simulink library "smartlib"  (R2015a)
settings: Solver=ode45  StartTime=0.0  StopTime=10.0  RelTol=1e-3
undefined symbols (not defined in the file or in its folder): annualChangeOfCostPerKwhFromUtility, batteryCostPerKwh, batterySize, compensationPerKwhSoldToBattery, costPerKwhBoughtFromBattery, costPerKwhFromUtility, csvread, numberOfHouses, oneTimeCost, randi, solarPanelEfficiency
libraries: simulink x7

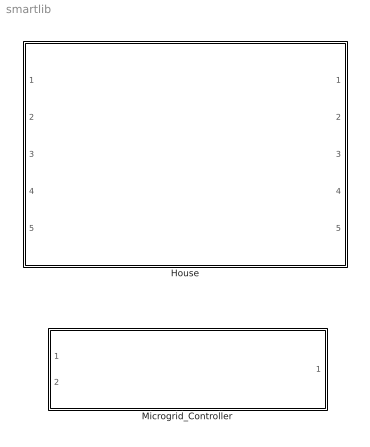
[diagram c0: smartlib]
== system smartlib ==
  House : Subsystem
  Microgrid_Controller : Subsystem

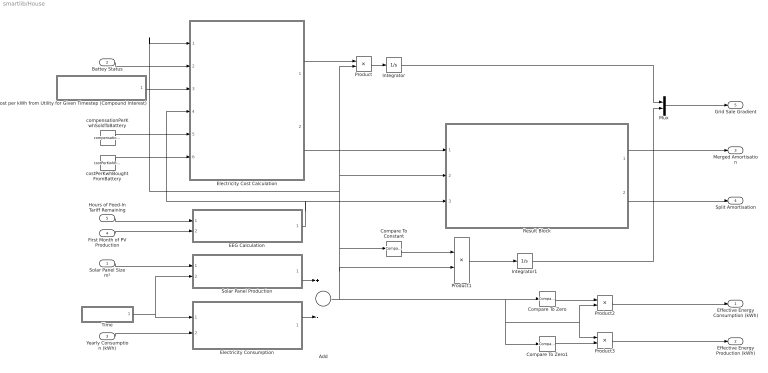
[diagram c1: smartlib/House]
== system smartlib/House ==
  Solar Panel Size m² : Inport
  Battey Status : Inport  Port=2
  Yearly Consumption (kWh) : Inport  Port=3
  First Month of PV Production : Inport  Port=4
  Hours of Feed-In Tariff Remaining : Inport  Port=5
  Add : Sum  Inputs=+-
  Compare To Constant : simulink/Logic and Bit Operations/Compare To Constant  relop=>=  const=0  OutDataTypeStr=boolean
  Compare To Zero : simulink/Logic and Bit Operations/Compare To Zero  relop=<  OutDataTypeStr=boolean
  Compare To Zero1 : simulink/Logic and Bit Operations/Compare To Zero  relop=>=  OutDataTypeStr=boolean
  Cost per kWh from Utility for Given Timestep (Compound Interest) : Subsystem
  EEG Calculation : Subsystem
  Electricity Consumption : Subsystem
  Electricity Cost Calculation : MATLAB Function  TreatAsAtomicUnit=on
  Integrator : Integrator
  Integrator1 : Integrator
  Mux : Mux  Inputs=2
  Product{,1..3} (4 alike) : Product
  Result Block : Subsystem
  Solar Panel Production : Subsystem
  Time : Subsystem
  compensationPerKwhSoldToBattery : Constant  Value=compensationPerKwhSoldToBattery
  costPerKwhBoughtFromBattery : Constant  Value=costPerKwhBoughtFromBattery
  Effective Energy Consumption (kWh) : Outport
  Effective Energy Production (kWh) : Outport  Port=2
  Merged Amortisation : Outport  Port=3
  Split Amortisation : Outport  Port=4
  Grid Sale Gradient : Outport  Port=5
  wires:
  Time/1(Time in Hours % 8760) -> Solar Panel Production/2(Hour of Year), Electricity Consumption/1(Hour of Year)
  Solar Panel Size m²/1 -> Solar Panel Production/1(Solar Panel Size (m²))
  Yearly Consumption (kWh)/1 -> Electricity Consumption/2(Yearly Consumption (kWh))
  Product/1 -> Integrator/1
  Compare To Constant/1 -> Product1/1
  Product1/1 -> Integrator1/1
  Product2/1 -> Effective Energy Consumption (kWh)/1
  Product3/1 -> Effective Energy Production (kWh)/1
  Compare To Zero1/1 -> Product3/2
  Compare To Zero/1 -> Product2/1
  Battey Status/1 -> Electricity Cost Calculation/2(batteryStatus)
  costPerKwhBoughtFromBattery/1 -> Electricity Cost Calculation/6(internalBuyPrice)
  Cost per kWh from Utility for Given Timestep (Compound Interest)/1(Cost for kWh from Utility at Timestep) -> Electricity Cost Calculation/3(buyPrice)
  Electricity Cost Calculation/1(gridsaleAmount) -> Product/1
  Electricity Consumption/1(Consumtion kWh) -> Add/2
  Solar Panel Production/1(Solar Panel Production (kWh)) -> Add/1
  Add/1 -> Compare To Zero1/1, Product3/1, Product2/2, Compare To Zero/1, Product/2, Result Block/2(Effective Consumption / Production (kWh)), Electricity Cost Calculation/1(kWh), Compare To Constant/1, Product1/2
  EEG Calculation/1(Applcable Feed-In Tariff) -> Electricity Cost Calculation/4(sellPrice), Result Block/3(Applicable Feed-In Tariff (EUR))
  Result Block/1(House Result Merged) -> Merged Amortisation/1
  Result Block/2(House Result Split) -> Split Amortisation/1
  Integrator/1 -> Mux/1
  Integrator1/1 -> Mux/2
  Mux/1 -> Grid Sale Gradient/1
  Electricity Cost Calculation/2(cost) -> Result Block/1(Effective Cost of Electricity for Timestep (EUR))
  Hours of Feed-In Tariff Remaining/1 -> EEG Calculation/1(Hours of Feed-In Tariff Remaining)
  First Month of PV Production/1 -> EEG Calculation/2(First Month of PV Production)
  compensationPerKwhSoldToBattery/1 -> Electricity Cost Calculation/5(internalSellPrice)

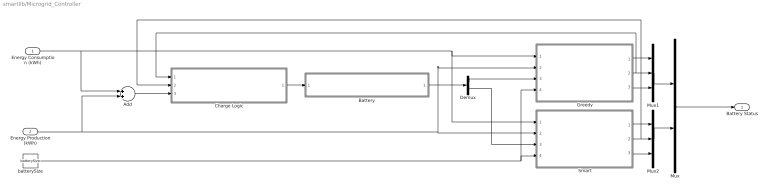
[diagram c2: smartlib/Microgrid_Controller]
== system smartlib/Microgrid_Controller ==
  Energy Consumption (kWh) : Inport
  Energy Production (kWh) : Inport  Port=2
  Add : Sum
  Battery : Subsystem
  Charge Logic : Subsystem
  Demux : Demux  Outputs=2
  Greedy : MATLAB Function  TreatAsAtomicUnit=on
  Mux : Mux  Inputs=2
  Mux1 : Mux  Inputs=3
  Mux2 : Mux  Inputs=3
  Smart : MATLAB Function  TreatAsAtomicUnit=on
  batterySize : Constant  Value=batterySize
  Battery Status : Outport
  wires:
  Charge Logic/1(Charge (kw/h)) -> Battery/1(Charge Amount (kWh))
  Mux/1 -> Battery Status/1
  batterySize/1 -> Smart/4(batterySize), Greedy/4(batterySize)
  Add/1 -> Charge Logic/3(Net Energy Amount (kWh))
  Demux/2 -> Smart/3(currentBatteryCharge)
  Demux/1 -> Greedy/3(currentBatteryCharge)
  Energy Consumption (kWh)/1 -> Greedy/1(Consumption), Smart/1(Consumption), Add/1
  Energy Production (kWh)/1 -> Smart/2(Production), Greedy/2(Production), Add/2
  Greedy/2(p2) -> Mux1/2, Charge Logic/1(Internal Trade Percentage - Greedy)
  Greedy/3(p3) -> Mux1/3
  Greedy/1(p1) -> Mux1/1
  Mux1/1 -> Mux/1
  Smart/1(p1) -> Mux2/1
  Smart/2(p2) -> Charge Logic/2(Internal Trade Percentage - Smart), Mux2/2
  Smart/3(p3) -> Mux2/3
  Mux2/1 -> Mux/2
  Battery/1(Current Battery Charge (kWh)) -> Demux/1

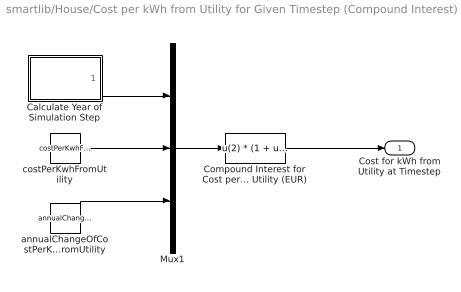
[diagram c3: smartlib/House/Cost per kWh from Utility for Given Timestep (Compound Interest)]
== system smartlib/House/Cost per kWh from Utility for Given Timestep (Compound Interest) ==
  Calculate Year of Simulation Step : Subsystem
  Compound Interest for Cost per kWh from Utility (EUR) : Fcn  Expr=u(2) * (1 + u(3) / 100) ^ u(1)
  Mux1 : Mux  Inputs=3
  annualChangeOfCostPerKwhFromUtility : Constant  Value=annualChangeOfCostPerKwhFromUtility
  costPerKwhFromUtility : Constant  Value=costPerKwhFromUtility
  Cost for kWh from Utility at Timestep : Outport
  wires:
  Mux1/1 -> Compound Interest for Cost per kWh from Utility (EUR)/1
  annualChangeOfCostPerKwhFromUtility/1 -> Mux1/3
  Calculate Year of Simulation Step/1(Out1) -> Mux1/1
  Compound Interest for Cost per kWh from Utility (EUR)/1 -> Cost for kWh from Utility at Timestep/1
  costPerKwhFromUtility/1 -> Mux1/2

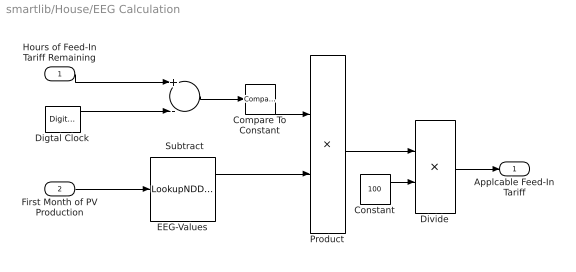
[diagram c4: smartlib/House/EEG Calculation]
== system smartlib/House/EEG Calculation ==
  Hours of Feed-In Tariff Remaining : Inport
  First Month of PV Production : Inport  Port=2
  Compare To Constant : simulink/Logic and Bit Operations/Compare To Constant  relop=>=  const=0  OutDataTypeStr=boolean
  Constant : Constant  Value=100
  Digtal Clock : DigitalClock
  Divide : Product  Inputs=*/
  EEG-Values : LookupNDDirect  NumberOfTableDimensions=1  Table=csvread('raw_data/feed-in_tariff_data.csv');  DiagnosticForOutOfRangeInput=Error
  Product : Product
  Subtract : Sum  Inputs=+-
  Applcable Feed-In Tariff : Outport
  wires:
  First Month of PV Production/1 -> EEG-Values/1
  Hours of Feed-In Tariff Remaining/1 -> Subtract/1
  Digtal Clock/1 -> Subtract/2
  Subtract/1 -> Compare To Constant/1
  Compare To Constant/1 -> Product/1
  EEG-Values/1 -> Product/2
  Divide/1 -> Applcable Feed-In Tariff/1
  Product/1 -> Divide/1
  Constant/1 -> Divide/2

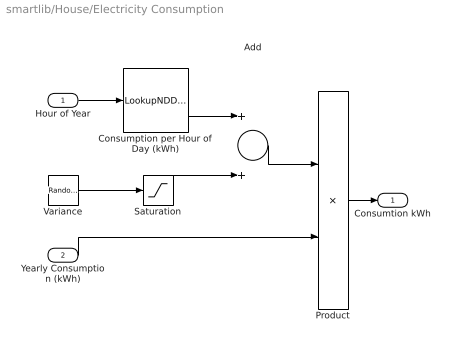
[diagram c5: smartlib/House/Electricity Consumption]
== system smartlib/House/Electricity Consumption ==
  Hour of Year : Inport
  Yearly Consumption (kWh) : Inport  Port=2
  Add : Sum
  Consumption per Hour of Day (kWh) : LookupNDDirect  NumberOfTableDimensions=1  Table=csvread('raw_data/netherlands_consumption_e1a.csv');  DiagnosticForOutOfRangeInput=Error
  Product : Product
  Saturation : Saturate  UpperLimit=5*10e-5  LowerLimit=-5*10e-5
  Variance : RandomNumber  Variance=0.00000000013014  Seed=randi(66666);  SampleTime=1
  Consumtion kWh : Outport
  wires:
  Add/1 -> Product/1
  Consumption per Hour of Day (kWh)/1 -> Add/1
  Hour of Year/1 -> Consumption per Hour of Day (kWh)/1
  Yearly Consumption (kWh)/1 -> Product/2
  Product/1 -> Consumtion kWh/1
  Variance/1 -> Saturation/1
  Saturation/1 -> Add/2

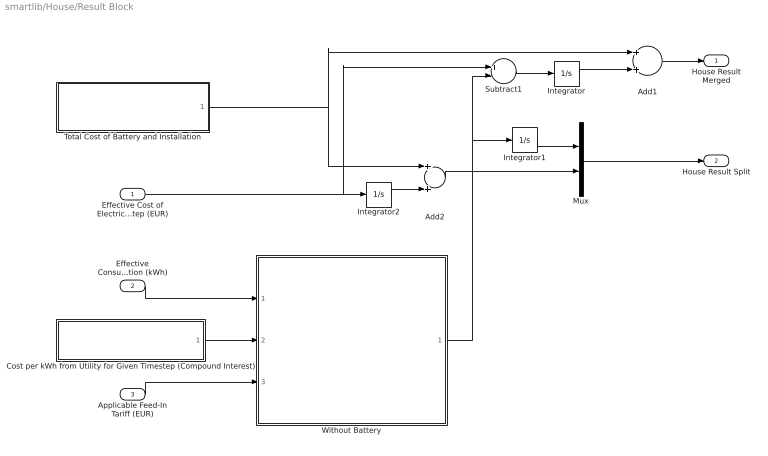
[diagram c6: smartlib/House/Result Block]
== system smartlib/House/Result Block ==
  Effective Cost of Electricity for Timestep (EUR) : Inport
  Effective Consumption / Production (kWh) : Inport  Port=2
  Applicable Feed-In Tariff (EUR) : Inport  Port=3
  Add1 : Sum
  Add2 : Sum
  Cost per kWh from Utility for Given Timestep (Compound Interest) : Subsystem
  Integrator : Integrator
  Integrator1 : Integrator
  Integrator2 : Integrator
  Mux : Mux  Inputs=2
  Subtract1 : Sum  Inputs=+-
  Total Cost of Battery and Installation : Subsystem
  Without Battery : Subsystem
  House Result Merged : Outport
  House Result Split : Outport  Port=2
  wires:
  Applicable Feed-In Tariff (EUR)/1 -> Without Battery/3(Sell Price to Utility (EUR))
  Subtract1/1 -> Integrator/1
  Effective Cost of Electricity for Timestep (EUR)/1 -> Subtract1/1, Integrator2/1
  Add1/1 -> House Result Merged/1
  Effective Consumption / Production (kWh)/1 -> Without Battery/1(Effective Consumption / Production (kWh))
  Integrator/1 -> Add1/2
  Mux/1 -> House Result Split/1
  Integrator1/1 -> Mux/1
  Integrator2/1 -> Add2/2
  Add2/1 -> Mux/2
  Total Cost of Battery and Installation/1(Total Cost of Battery and Installation) -> Add1/1, Add2/1
  Cost per kWh from Utility for Given Timestep (Compound Interest)/1(Cost per kWh from Utility at Timestep) -> Without Battery/2(Cost per kWh from Utility (EUR))
  Without Battery/1(Result EUR) -> Integrator1/1, Subtract1/2

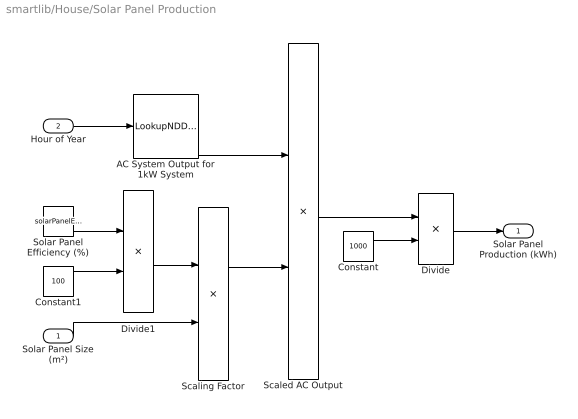
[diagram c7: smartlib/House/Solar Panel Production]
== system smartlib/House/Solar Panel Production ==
  Solar Panel Size (m²) : Inport
  Hour of Year : Inport  Port=2
  AC System Output for 1kW System : LookupNDDirect  NumberOfTableDimensions=1  Table=csvread('raw_data/pvwatts_data_1kwp.csv');  DiagnosticForOutOfRangeInput=Error
  Constant : Constant  Value=1000
  Constant1 : Constant  Value=100
  Divide : Product  Inputs=*/
  Divide1 : Product  Inputs=*/
  Scaled AC Output : Product
  Scaling Factor : Product
  Solar Panel Efficiency (%) : Constant  Value=solarPanelEfficiency
  Solar Panel Production (kWh) : Outport
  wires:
  Solar Panel Efficiency (%)/1 -> Divide1/1
  Scaling Factor/1 -> Scaled AC Output/2
  AC System Output for 1kW System/1 -> Scaled AC Output/1
  Solar Panel Size (m²)/1 -> Scaling Factor/2
  Hour of Year/1 -> AC System Output for 1kW System/1
  Scaled AC Output/1 -> Divide/1
  Constant/1 -> Divide/2
  Divide/1 -> Solar Panel Production (kWh)/1
  Constant1/1 -> Divide1/2
  Divide1/1 -> Scaling Factor/1

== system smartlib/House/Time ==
  Digtal Clock : DigitalClock
  Hours in a Year : Constant  Value=8760
  Modulo : Math  Operator=mod
  Time in Hours % 8760 : Outport
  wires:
  Digtal Clock/1 -> Modulo/1
  Hours in a Year/1 -> Modulo/2
  Modulo/1 -> Time in Hours % 8760/1

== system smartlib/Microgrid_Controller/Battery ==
  Charge Amount (kWh) : Inport
  Battery : Integrator
  To Workspace : ToWorkspace  VariableName=neighbourhood_battery_charge_over_time  SaveFormat=Timeseries  SampleTime=-1
  Current Battery Charge (kWh) : Outport
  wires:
  Battery/1 -> Current Battery Charge (kWh)/1, To Workspace/1
  Charge Amount (kWh)/1 -> Battery/1

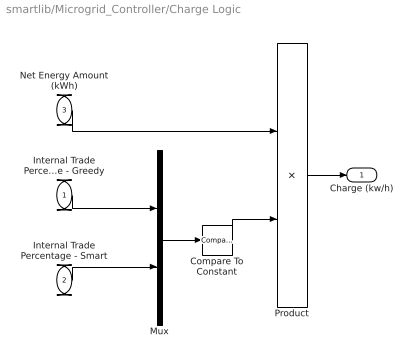
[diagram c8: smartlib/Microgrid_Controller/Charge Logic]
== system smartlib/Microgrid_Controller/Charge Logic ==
  Internal Trade Percentage - Greedy : Inport
  Internal Trade Percentage - Smart : Inport  Port=2
  Net Energy Amount (kWh) : Inport  Port=3
  Compare To Constant : simulink/Logic and Bit Operations/Compare To Constant  relop===  const=1  OutDataTypeStr=boolean
  Mux : Mux  Inputs=2
  Product : Product
  Charge (kw/h) : Outport
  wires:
  Net Energy Amount (kWh)/1 -> Product/1
  Product/1 -> Charge (kw/h)/1
  Internal Trade Percentage - Greedy/1 -> Mux/1
  Mux/1 -> Compare To Constant/1
  Internal Trade Percentage - Smart/1 -> Mux/2
  Compare To Constant/1 -> Product/2

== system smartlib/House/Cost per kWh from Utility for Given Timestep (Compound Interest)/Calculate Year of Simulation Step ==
  Digital Clock : DigitalClock
  Fcn : Fcn  Expr=floor(u/8760)
  Out1 : Outport
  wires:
  Fcn/1 -> Out1/1
  Digital Clock/1 -> Fcn/1

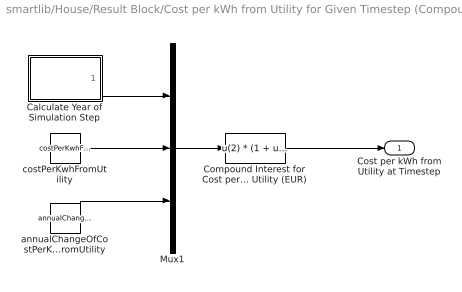
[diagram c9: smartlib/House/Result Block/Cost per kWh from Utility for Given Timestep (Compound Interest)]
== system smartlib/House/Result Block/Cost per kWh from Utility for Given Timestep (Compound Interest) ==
  Calculate Year of Simulation Step : Subsystem
  Compound Interest for Cost per kWh from Utility (EUR) : Fcn  Expr=u(2) * (1 + u(3) / 100) ^ u(1)
  Mux1 : Mux  Inputs=3
  annualChangeOfCostPerKwhFromUtility : Constant  Value=annualChangeOfCostPerKwhFromUtility
  costPerKwhFromUtility : Constant  Value=costPerKwhFromUtility
  Cost per kWh from Utility at Timestep : Outport
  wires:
  Mux1/1 -> Compound Interest for Cost per kWh from Utility (EUR)/1
  annualChangeOfCostPerKwhFromUtility/1 -> Mux1/3
  Calculate Year of Simulation Step/1(Out1) -> Mux1/1
  Compound Interest for Cost per kWh from Utility (EUR)/1 -> Cost per kWh from Utility at Timestep/1
  costPerKwhFromUtility/1 -> Mux1/2

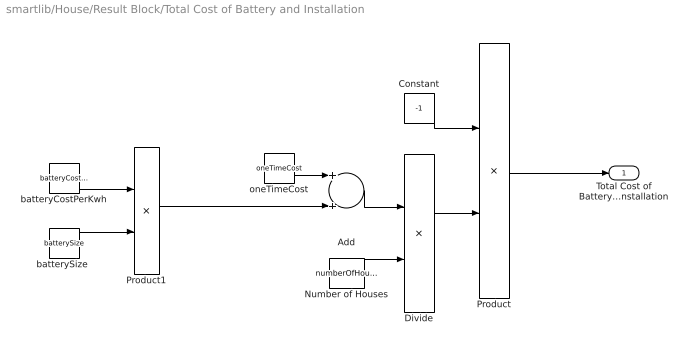
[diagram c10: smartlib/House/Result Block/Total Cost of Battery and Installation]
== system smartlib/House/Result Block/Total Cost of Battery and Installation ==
  Add : Sum
  Constant : Constant  Value=-1
  Divide : Product  Inputs=*/
  Number of Houses : Constant  Value=numberOfHouses
  Product : Product
  Product1 : Product
  batteryCostPerKwh : Constant  Value=batteryCostPerKwh
  "batterySize " : Constant  Value=batterySize
  oneTimeCost : Constant  Value=oneTimeCost
  Total Cost of Battery and Installation : Outport
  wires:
  Constant/1 -> Product/1
  oneTimeCost/1 -> Add/1
  Number of Houses/1 -> Divide/2
  Add/1 -> Divide/1
  Divide/1 -> Product/2
  "batterySize "/1 -> Product1/2
  Product/1 -> Total Cost of Battery and Installation/1
  batteryCostPerKwh/1 -> Product1/1
  Product1/1 -> Add/2

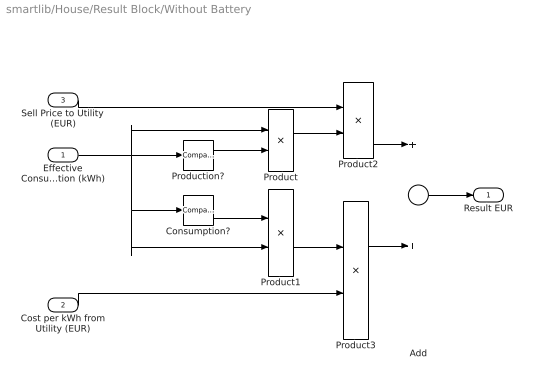
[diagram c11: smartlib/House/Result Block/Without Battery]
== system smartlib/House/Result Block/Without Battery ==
  Effective Consumption / Production (kWh) : Inport
  Cost per kWh from Utility (EUR) : Inport  Port=2
  Sell Price to Utility (EUR) : Inport  Port=3
  Add : Sum
  Consumption? : simulink/Logic and Bit Operations/Compare To Zero  relop=<  OutDataTypeStr=boolean
  Product{,1..3} (4 alike) : Product
  Production? : simulink/Logic and Bit Operations/Compare To Zero  relop=>=  OutDataTypeStr=boolean
  Result EUR : Outport
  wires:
  Effective Consumption / Production (kWh)/1 -> Product/1, Product1/2, Consumption?/1, Production?/1
  Consumption?/1 -> Product1/1
  Production?/1 -> Product/2
  Product/1 -> Product2/2
  Sell Price to Utility (EUR)/1 -> Product2/1
  Product1/1 -> Product3/1
  Cost per kWh from Utility (EUR)/1 -> Product3/2
  Product3/1 -> Add/2
  Product2/1 -> Add/1
  Add/1 -> Result EUR/1

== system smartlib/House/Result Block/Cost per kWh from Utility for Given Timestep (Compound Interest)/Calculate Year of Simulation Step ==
  Digital Clock : DigitalClock
  Fcn : Fcn  Expr=floor(u/8760)
  Out1 : Outport
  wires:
  Fcn/1 -> Out1/1
  Digital Clock/1 -> Fcn/1

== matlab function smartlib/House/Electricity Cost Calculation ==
function [gridsaleAmount, cost]  = costCalculation(kWh, batteryStatus, buyPrice, sellPrice, internalSellPrice, internalBuyPrice)


cost = zeros(numel(batteryStatus)/3 , 1);
gridsaleAmount = zeros(numel(batteryStatus)/3 , 1);


for i = 1:numel(cost)
    
    %Production?
    
    if (kWh >= 0)
        
        cost(i) = kWh * sellPrice * batteryStatus((i-1)*3+1) + kWh * internalSellPrice * (batteryStatus((i-1)*3+2)+batteryStatus((i-1)*3+3));
        gridsaleAmount(i) = batteryStatus((i-1)*3+1);
        
    %Consumption?
    
    else
        
        cost(i) = kWh * buyPrice * batteryStatus((i-1)*3+3) + kWh * internalBuyPrice * (batteryStatus((i-1)*3+1)+batteryStatus((i-1)*3+2));
        gridsaleAmount(i) = 0;
        
    end
    
end

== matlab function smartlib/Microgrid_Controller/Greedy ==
function [p1,p2,p3]  = fcn(Consumption, Production, currentBatteryCharge, batterySize)
%fcn computes ???
%   Detailed desciription

p1 = 0;
p2 = 1;
p3 = 0;

Consumption = -Consumption;

% "Status" = aktueller Füllstand
% "Size" = Größe der Batterie in kWh

%Energie verkaufen
% Heißt "Strom muss an das externe Netz verkauft werden, falls die Batterie
% voll ist"?
if (currentBatteryCharge >= batterySize && Production ~= 0 && Consumption < Production)
    
    p2 = Consumption / Production;
    p1 = 1 - p2;
    
end

%Energie einkaufen
if (currentBatteryCharge <= 0 && Consumption ~= 0 && Consumption > Production)
    
    p2 = Production / Consumption;
    p3 = 1 - p2;
    
end

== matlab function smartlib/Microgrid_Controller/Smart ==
function [p1,p2,p3]  = fcn(Consumption, Production, currentBatteryCharge, batterySize)
%fcn computes ???
%   Detailed desciription

p1 = 0;
p2 = 1;
p3 = 0;

smart = 0.3;

Consumption = -Consumption;

% "Status" = aktueller Füllstand
% "Size" = Größe der Batterie in kWh

%Energie verkaufen
% Heißt "Strom muss an das externe Netz verkauft werden, falls die Batterie
% voll ist"?
if (currentBatteryCharge >= batterySize && Production ~= 0 && Consumption < Production)
    
    p2 = Consumption / Production;
    p1 = 1 - p2;
    
end

%Energie einkaufen
if (currentBatteryCharge <= batterySize * 0.3 && Consumption ~= 0 && Consumption > Production)
    
    p2 = Production / Consumption;
    p3 = 1 - p2;
    
end
